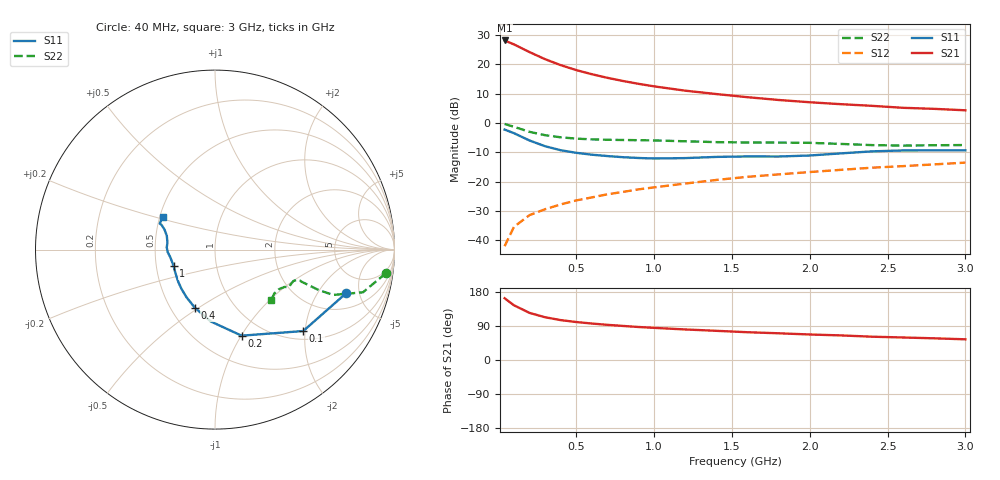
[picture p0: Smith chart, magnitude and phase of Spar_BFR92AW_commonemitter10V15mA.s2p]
! Filename:  BFR92AWI.S2P  Version:  4.0
! NXP part #: BFR92AW  Date: Jun 1994
! Bias condition: Vce=10V, Ic=15mA
#  MHz  S  MA  R  50
! Freq  S11  S21  S12  S22  !GUM [dB]
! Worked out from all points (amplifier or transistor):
!   21 points, 40 MHz to 3 GHz, reference 50 ohm
!   highest |S21| = 28.1 dB at 40 MHz (marker M1)
!   |S21| within 3 dB of that: start of sweep to 163.5 MHz
!   unconditionally stable (mu >= 1): 634.7 MHz to end of sweep
!   at 300 MHz: K = 0.75, MSG = 25.5 dB, |S12| = -29.4 dB
!   at 1 GHz: K = 1.10, MAG = 15.2 dB, |S12| = -21.9 dB
!   at 3 GHz: K = 1.09, MAG = 7.0 dB, |S12| = -13.5 dB
!   lowest NFmin = 2.30 dB at 500 MHz
!   S11 on the Smith chart (normalised r, x): 40 MHz: 3.09, -3.69; 100 MHz: 1.19, -1.95; 200 MHz: 0.78, -1.00; 400 MHz: 0.66, -0.48; 1 GHz: 0.62, -0.12; 3 GHz: 0.52, +0.21
40  0.77 -18.4  25.27 163.0  0.008 80.7  0.961 -7.9
100  0.669 -42.7  21.66 144.4  0.017 70.1  0.858 -16.1
200  0.502 -72.8  16.02 124.3  0.027 63.1  0.705 -21.0
300  0.401 -93.4  12.13 112.8  0.034 62.4  0.618 -21.3
400  0.343 -109.0  9.616 105.3  0.041 63.8  0.569 -20.9
500  0.31 -120.6  7.917 100.2  0.048 65.4  0.54 -20.6
600  0.288 -130.4  6.737 96.2  0.054 67.2  0.525 -20.5
700  0.273 -138.3  5.849 92.8  0.061 68.6  0.517 -20.4
800  0.261 -145.5  5.169 89.9  0.067 69.8  0.512 -20.3
900  0.253 -152.3  4.624 87.1  0.074 70.6  0.508 -20.1
1000  0.248 -158.7  4.185 84.8  0.08 71.4  0.503 -20.0
1200  0.252 -169.6  3.535 80.6  0.093 72.3  0.487 -20.2
1400  0.264 -177.0  3.097 77.0  0.107 73.1  0.471 -21.8
1600  0.269 177.6  2.739 73.3  0.121 73.5  0.464 -24.6
1800  0.268 171.6  2.455 70.5  0.133 74.1  0.463 -26.2
2000  0.279 164.1  2.246 67.3  0.146 74.5  0.458 -27.1
2200  0.303 158.3  2.082 64.9  0.159 74.8  0.439 -28.3
2400  0.328 155.2  1.951 61.5  0.173 74.8  0.419 -31.8
2600  0.34 154.8  1.806 59.4  0.184 74.8  0.411 -36.6
2800  0.341 152.5  1.734 57.2  0.197 75.5  0.417 -40.1
3000  0.342 147.9  1.639 54.6  0.211 75.6  0.42 -42.0
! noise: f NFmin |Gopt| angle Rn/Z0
500  2.3  0.35  18.8  0.47
1000  2.8  0.252  47.3  0.49
2000  3.7  0.166  173  0.33
